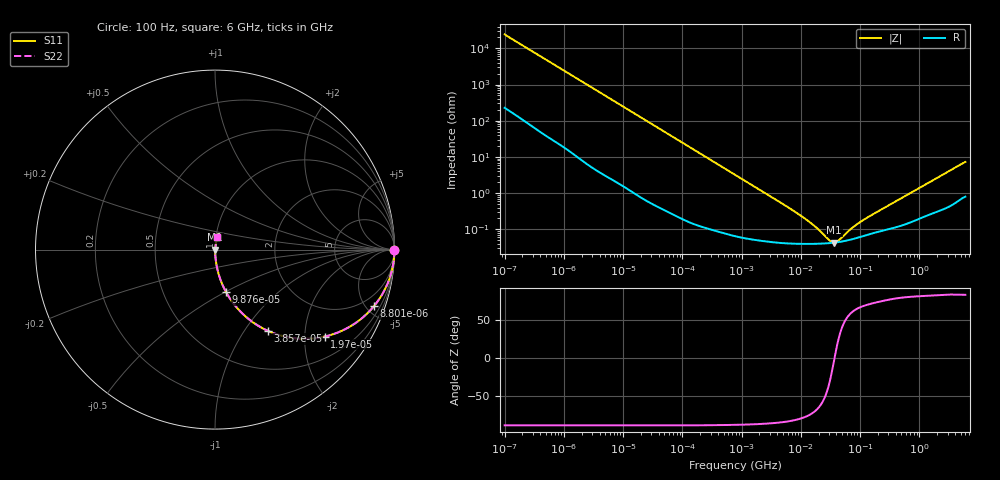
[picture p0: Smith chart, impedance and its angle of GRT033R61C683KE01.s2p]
!Murata Part Number: GRT033R61C683KE01
!These Parameters are Measured in Series Mode Connection
!Data Generated on Jun 19, 2026
!  o--ll--o
!Port1  Port2
!  o------o
!Operation Temp=25[degC], DC Bias Voltage=0[V]
!Freq. Start=100[Hz] Stop=6[GHz] 401[Steps]
# Hz S RI R 50
!Freq.(Hz) S11(Real) S11(Imag) S21(Real) S21(Imag) S12(Real) S12(Imag) S22(Real) S22(Imag)
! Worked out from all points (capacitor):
!   401 points, 100 Hz to 6 GHz, reference 50 ohm
!   read as one part in series: C = 65.9 nF near 109 Hz
!   lowest |Z| = 43 mohm at 36.42 MHz (marker M1)
!   series resonance near 37.12 MHz, so ESL is about 280 pH
!   S11 on the Smith chart (normalised r, x): 100 Hz: open; 8.801 kHz: 1.04, -5.60; 19.7 kHz: 1.02, -2.51; 38.57 kHz: 1.01, -1.28; 98.76 kHz: 1.00, -0.50; 6 GHz: 1.02, +0.14
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100  0.9999 -0.00415  5.62e-05 0.00415  5.62e-05 0.00415  0.9999 -0.00415
627  0.9991 -0.0257  0.000862 0.0257  0.000862 0.0257  0.9991 -0.0257
2008  0.9928 -0.0813  0.00721 0.0813  0.00721 0.0813  0.9928 -0.0813
4918  0.9604 -0.192  0.0396 0.192  0.0396 0.192  0.9604 -0.192
8801  0.8852 -0.3156  0.1148 0.3156  0.1148 0.3156  0.8852 -0.3156
13169  0.7768 -0.4133  0.2232 0.4133  0.2232 0.4133  0.7768 -0.4133
19704  0.6105 -0.4846  0.3895 0.4846  0.3895 0.4846  0.6105 -0.4846
26957  0.4572 -0.4951  0.5428 0.4951  0.5428 0.4951  0.4572 -0.4951
38569  0.293 -0.4519  0.707 0.4519  0.707 0.4519  0.293 -0.4519
40335  0.275 -0.4433  0.725 0.4433  0.725 0.4433  0.275 -0.4433
60352  0.1462 -0.3498  0.8538 0.3498  0.8538 0.3498  0.1462 -0.3498
98762  0.0611 -0.2357  0.9389 0.2357  0.9389 0.2357  0.0611 -0.2357
241822  0.0116 -0.1018  0.9884 0.1018  0.9884 0.1018  0.0116 -0.1018
774597  0.00169 -0.0323  0.9983 0.0323  0.9983 0.0323  0.00169 -0.0323
6353432  0.000421 -0.00387  0.9996 0.00387  0.9996 0.00387  0.000421 -0.00387
1.555665e7  0.000399 -0.00134  0.9996 0.00134  0.9996 0.00134  0.000399 -0.00134
3.045065e7  0.000417 -0.00027  0.9996 0.00027  0.9996 0.00027  0.000417 -0.00027
3.64232e7  0.000429 -2.53e-05  0.9996 2.53e-05  0.9996 2.53e-05  0.000429 -2.53e-05
4.35672e7  0.000446 0.000216  0.9996 -0.000216  0.9996 -0.000216  0.000446 0.000216
9.753859e7  0.000609 0.00141  0.9994 -0.00141  0.9994 -0.00141  0.000609 0.00141
3.124326e8  0.00104 0.00457  0.999 -0.00457  0.999 -0.00457  0.00104 0.00457
6e9  0.013 0.0709  0.987 -0.0709  0.987 -0.0709  0.013 0.0709
